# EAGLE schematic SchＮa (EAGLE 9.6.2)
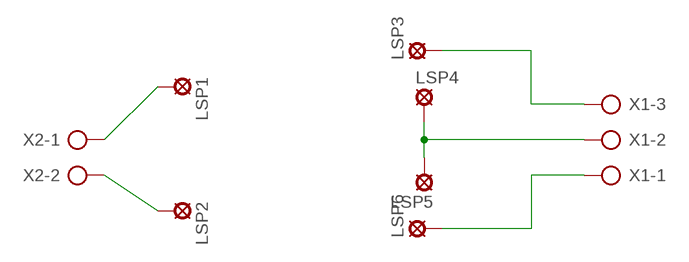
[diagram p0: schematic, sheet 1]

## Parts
LSP1  LSP10  [LSP10]
LSP2  LSP10  [LSP10]
LSP3  LSP10  [LSP10]
LSP4  LSP10  [LSP10]
LSP5  LSP10  [LSP10]
LSP6  LSP10  [LSP10]
X1  AK500/3  [AK500/3]
X2  AK500/2  [AK500/2]

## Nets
N$1: LSP4.MP LSP5.MP X1.2
N$2: LSP3.MP X1.3
N$3: LSP6.MP X1.1
N$4: LSP1.MP X2.1
N$5: LSP2.MP X2.2

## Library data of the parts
LSP1-LSP6 = solpad:LSP10: SOLDER PAD
X1 = con-ptr500:AK500/3: CONNECTOR; OC_FARNELL: unknown; OC_NEWARK: unknown
X2 = con-ptr500:AK500/2: CONNECTOR; OC_FARNELL: unknown; OC_NEWARK: unknown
